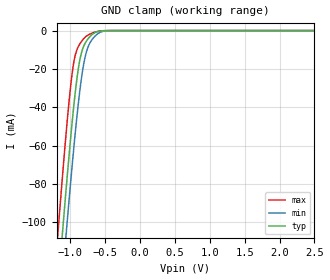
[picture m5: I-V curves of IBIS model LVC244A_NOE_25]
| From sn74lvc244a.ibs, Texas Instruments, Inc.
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[Model]   LVC244A_NOE_25
Model_type  Input
Vinl=0.7
Vinh=1.7
| variable   typ   min   max
C_comp   2.58pF   2.07pF   3.26pF
[Temperature Range]   40   100   -40
| Ambient temperature   25   85   -40
[Voltage range]   2.5   2.3   2.7
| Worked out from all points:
|   GND clamp passes 1 mA (typ) near -0.64 V on its own axis
[GND Clamp]
| LVC244A_NOE_25
|   Voltage   I(typ)   I(min)   I(max)
-5.5V     -2.303A    -2.296A    -2.31A
-1.18V    -134.8mA   -158.2mA   -105.7mA
-1.12V    -107.8mA   -131.4mA   -78.37mA
-1.07V    -85.97mA   -109.6mA   -56.7mA
-1.055V   -79.59mA   -103.1mA   -50.5mA
-965mV    -43.83mA   -66.22mA   -19.51mA
-925mV    -30.3mA    -51.14mA   -12.01mA
-865mV    -15.24mA   -31.21mA   -6.925mA
-810mV    -8.148mA   -17.45mA   -4.19mA
-765mV    -5.168mA   -10.4mA    -2.744mA
-625mV    -729.3uA   -2.13mA    -560.8uA
2.5V      57.25pA    177pA      32.61pA
